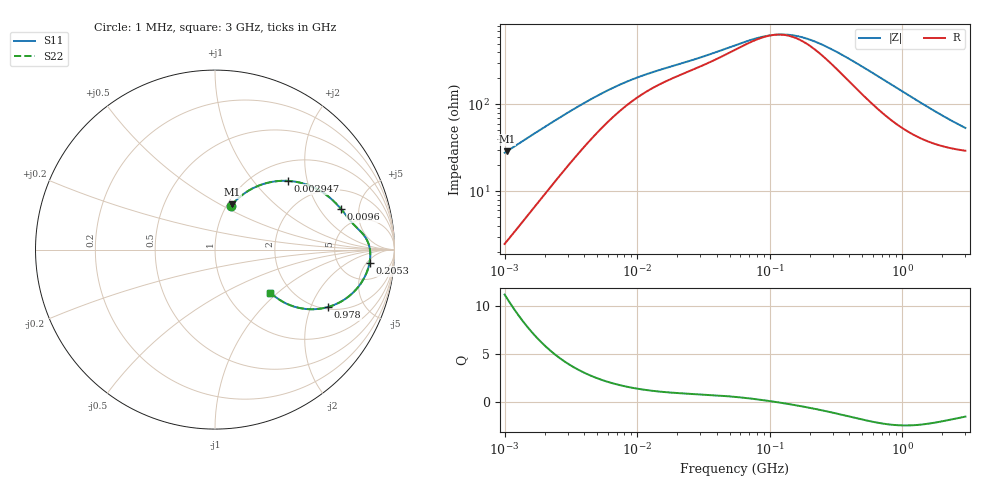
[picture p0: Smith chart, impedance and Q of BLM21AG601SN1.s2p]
! BLM21AG601SN1
# Hz S RI R 50
!Freq.(Hz) S11(Real) S11(Imag) S21(Real) S21(Imag) S12(Real) S12(Imag) S22(Real) S22(Imag)
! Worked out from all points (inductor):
!   401 points, 1 MHz to 3 GHz, reference 50 ohm
!   read as one part in series: L = 4.36 uH near 1.041 MHz
!   highest Q = 10.8 at 1.041 MHz (marker M1), where L = 4.38 uH
!   self-resonance near 110.1 MHz
!   S11 on the Smith chart (normalised r, x): 1 MHz: 1.05, +0.55; 2.947 MHz: 1.38, +1.53; 9.6 MHz: 3.28, +3.24; 205.3 MHz: 10, -6; 978 MHz: 2.09, -2.67; 3 GHz: 1.58, -0.89
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1000000  0.0898 0.2447  0.9102 -0.2447  0.9102 -0.2447  0.0898 0.2447
1040844  0.0963 0.2523  0.9037 -0.2523  0.9037 -0.2523  0.0963 0.2523
1682724  0.2075 0.3399  0.7925 -0.3399  0.7925 -0.3399  0.2075 0.3399
2271982  0.3081 0.3756  0.6919 -0.3756  0.6919 -0.3756  0.3081 0.3756
2947212  0.4053 0.3829  0.5947 -0.3829  0.5947 -0.3829  0.4053 0.3829
3823119  0.499 0.3662  0.501 -0.3662  0.501 -0.3662  0.499 0.3662
5938264  0.6233 0.3023  0.3767 -0.3023  0.3767 -0.3023  0.6233 0.3023
9600343  0.7033 0.2247  0.2967 -0.2247  0.2967 -0.2247  0.7033 0.2247
1.461624e7  0.744 0.173  0.256 -0.173  0.256 -0.173  0.744 0.173
5.477226e7  0.8379 0.0684  0.1621 -0.0684  0.1621 -0.0684  0.8379 0.0684
8.338914e7  0.8567 0.0288  0.1433 -0.0288  0.1433 -0.0288  0.8567 0.0288
1.125904e8  0.8637 -0.00239  0.1363 0.00239  0.1363 0.00239  0.8637 -0.00239
1.520175e8  0.8652 -0.0362  0.1348 0.0362  0.1348 0.0362  0.8652 -0.0362
2.052512e8  0.8609 -0.0738  0.1391 0.0738  0.1391 0.0738  0.8609 -0.0738
2.094008e8  0.8604 -0.0765  0.1396 0.0765  0.1396 0.0765  0.8604 -0.0765
4.391493e8  0.8089 -0.1938  0.1911 0.1938  0.1911 0.1938  0.8089 -0.1938
5.929311e8  0.7602 -0.2482  0.2398 0.2482  0.2398 0.2482  0.7602 -0.2482
8.005644e8  0.6888 -0.2969  0.3112 0.2969  0.3112 0.2969  0.6888 -0.2969
9.779672e8  0.6293 -0.32  0.3707 0.32  0.3707 0.32  0.6293 -0.32
1.581072e9  0.4702 -0.3252  0.5298 0.3252  0.5298 0.3252  0.4702 -0.3252
2.221924e9  0.372 -0.2872  0.628 0.2872  0.628 0.2872  0.372 -0.2872
3e9  0.3087 -0.2394  0.6913 0.2394  0.6913 0.2394  0.3087 -0.2394
